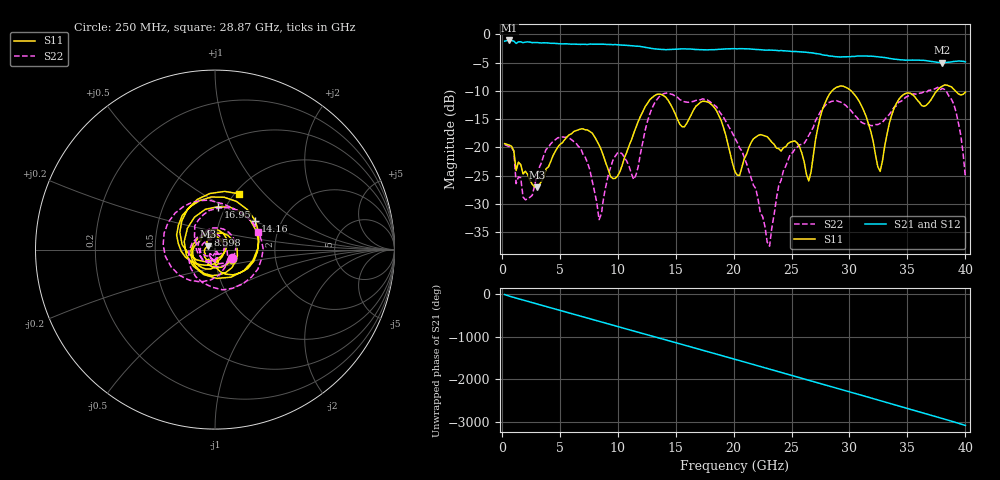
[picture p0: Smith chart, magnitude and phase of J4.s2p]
!Agilent Technologies,E8364B,MY43040528,A.07.50.67
!Agilent E8364B: A.07.50.67
!Date: Thursday, May 22, 2025 21:07:32
!Correction: S11(Full 2 Port(1,2))
!S21(Full 2 Port(1,2))
!S12(Full 2 Port(1,2))
!S22(Full 2 Port(1,2))
!S2P File: Measurements: S11, S21, S12, S22:
# Hz S  dB  R 50
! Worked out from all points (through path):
!   201 points, 250 MHz to 40 GHz, reference 50 ohm
!   highest |S21| = -1.11 dB at 647.5 MHz (marker M1); lowest = -5.1 dB at 38.01 GHz (marker M2)
!   group delay of S21, straight-line fit = 213 ps
!   lowest |S11| = -27.0 dB at 3.033 GHz (marker M3), VSWR 1.09, Z = 46.1 + j1.69 ohm
!   |S11| at or under -10 dB: start of sweep to 28.51 GHz; 30.14 GHz to 37.54 GHz (7.405 GHz wide, 21.9 % of centre); 39.13 GHz to end of sweep
!   |S22| runs from -37.4 to -9.4 dB; largest |S21 - S12| = 0.0075
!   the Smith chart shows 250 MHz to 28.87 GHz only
!   S11 on the Smith chart (normalised r, x): 250 MHz: 1.20, -0.13; 8.598 GHz: 0.91, +0.15; 14.16 GHz: 1.47, +0.52; 16.95 GHz: 0.92, +0.47; 28.87 GHz: 1.05, +0.74
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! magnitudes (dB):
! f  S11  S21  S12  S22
! 250 MHz  -19.3  -1.2  -1.3  -19.5
! 647.5 MHz  -19.6  -1.1  -1.1  -19.9
! 2.039 GHz  -24.2  -1.4  -1.4  -29.2
! 3.033 GHz  -27.0  -1.5  -1.5  -24.9
! 7.008 GHz  -16.7  -1.8  -1.8  -21.2
! 8.598 GHz  -20.5  -1.8  -1.8  -31.8
! 9.989 GHz  -25.1  -1.9  -1.9  -21.0
! 11.38 GHz  -17.6  -2.1  -2.1  -25.7
! 13.57 GHz  -10.6  -2.7  -2.7  -11.1
! 14.16 GHz  -11.2  -2.7  -2.7  -10.4
! 16.95 GHz  -12.4  -2.7  -2.7  -11.6
! 20.12 GHz  -24.3  -2.6  -2.6  -18.4
! 23.11 GHz  -18.6  -2.8  -2.9  -37.4
! 24.3 GHz  -20.0  -2.9  -2.9  -24.1
! 26.88 GHz  -21.4  -3.3  -3.3  -16.4
! 28.87 GHz  -9.4  -4.0  -4.0  -11.7
! 31.06 GHz  -12.7  -3.8  -3.9  -15.6
! 32.65 GHz  -24.2  -4.0  -4.1  -15.7
! 33.44 GHz  -15.7  -4.3  -4.3  -14.2
! 38.01 GHz  -9.2  -5.1  -5.1  -9.6
! 39.2 GHz  -10.2  -4.8  -4.8  -13.8
! 40 GHz  -10.2  -4.9  -4.9  -25.3
